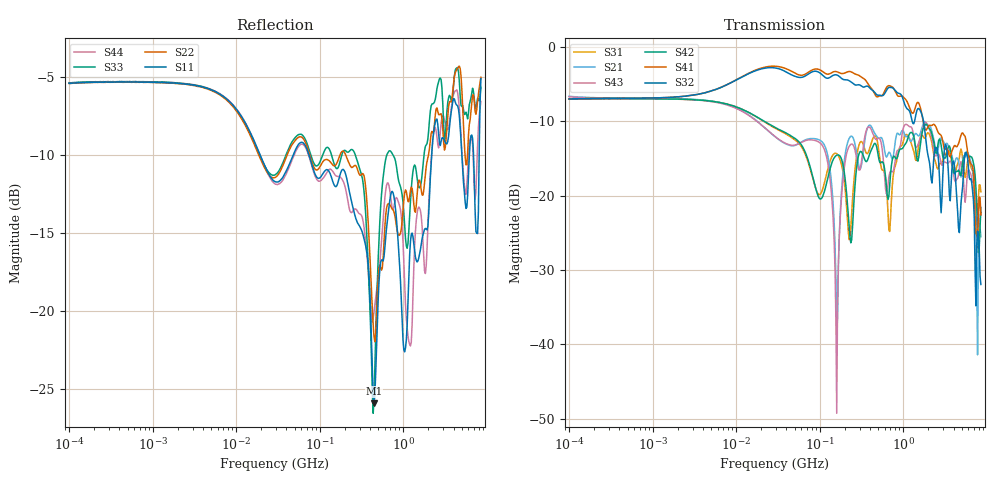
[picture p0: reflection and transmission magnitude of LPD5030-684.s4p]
# MHz S MA R 50
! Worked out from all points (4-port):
!   498 points, 100 kHz to 8.5 GHz, reference 50 ohm
!   strongest paths, dB at 100 kHz, 1.698 MHz, 29.49 MHz, 500.7 MHz, 8.5 GHz:
!     S32: -7.0, -6.8, -2.8, -6.5, -31.9
!     S41: -7.0, -6.8, -2.6, -6.7, -22.6
!     S42: -7.0, -7.0, -10.8, -14.6, -21.6
!     S43: -6.7, -7.0, -12.1, -12.3, -22.2
!     S21: -6.6, -6.9, -12.1, -12.2, -25.5
!     S31: -7.0, -7.0, -10.9, -13.3, -19.5
!   lowest |S11| = -25.9 dB at 446.6 MHz (marker M1), VSWR 1.11, Z = 51.9 - j4.79 ohm
!   |S11| at or under -10 dB: 74.1 MHz to 2.192 GHz (2.118 GHz wide, 187 % of centre); 5.028 GHz to 6.193 GHz (1.165 GHz wide, 20.8 % of centre); 6.936 GHz to 8.106 GHz (1.171 GHz wide, 15.6 % of centre)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
0.1  0.5357 6.1  0.4669 -8.0  0.4466 -172.8  0.4487 8.0
     0.4669 -8.0  0.5346 6.1  0.4478 8.0  0.447 -172.9
     0.4466 -172.8  0.4478 8.0  0.5375 6.2  0.4639 -8.0
     0.4487 8.0  0.447 -172.9  0.4639 -8.0  0.5364 6.1
101.2184  0.2669 -27.6  0.236 45.8  0.102 -158.3  0.7017 -19.8
          0.236 45.8  0.2899 -19.5  0.6684 -23.0  0.09504 -155.3
          0.102 -158.3  0.6684 -23.0  0.3005 -17.2  0.2264 45.2
          0.7017 -19.8  0.09504 -155.3  0.2264 45.2  0.2605 -26.1
159.8183  0.2511 -36.4  0.01207 -113.6  0.1918 46.1  0.6831 -29.6
          0.01207 -113.6  0.2965 -27.0  0.6495 -33.1  0.1874 50.3
          0.1918 46.1  0.6495 -33.1  0.285 -29.5  0.003442 26.5
          0.6831 -29.6  0.1874 50.3  0.003442 26.5  0.2697 -38.5
446.6343  0.05049 -65.8  0.2681 -35.5  0.2511 -36.2  0.4953 -82.7
          0.2681 -35.5  0.08249 -77.2  0.5022 -80.8  0.2226 -28.5
          0.2511 -36.2  0.5022 -80.8  0.05164 -34.0  0.2505 -42.0
          0.4953 -82.7  0.2226 -28.5  0.2505 -42.0  0.09884 -54.3
2776.003  0.3381 16.9  0.2445 1.5  0.1662 -3.5  0.2582 -30.8
          0.2445 1.5  0.4261 19.5  0.0968 -51.7  0.2348 -16.8
          0.1662 -3.5  0.0968 -51.7  0.5568 12.2  0.1767 -15.1
          0.2582 -30.8  0.2348 -16.8  0.1767 -15.1  0.3731 32.6
4484.409  0.4526 178.6  0.177 133.8  0.1643 137.8  0.218 130.1
          0.177 133.8  0.5975 -178.0  0.0775 103.2  0.1462 128.5
          0.1643 137.8  0.0775 103.2  0.5989 170.4  0.131 143.9
          0.218 130.1  0.1462 128.5  0.131 143.9  0.4984 174.8
8500  0.5542 -18.5  0.05308 30.2  0.1063 -18.9  0.07429 -43.4
      0.05308 30.2  0.5597 -34.3  0.02533 3.4  0.08348 7.8
      0.1063 -18.9  0.02533 3.4  0.5201 -40.3  0.07782 15.1
      0.07429 -43.4  0.08348 7.8  0.07782 15.1  0.4681 -39.9
